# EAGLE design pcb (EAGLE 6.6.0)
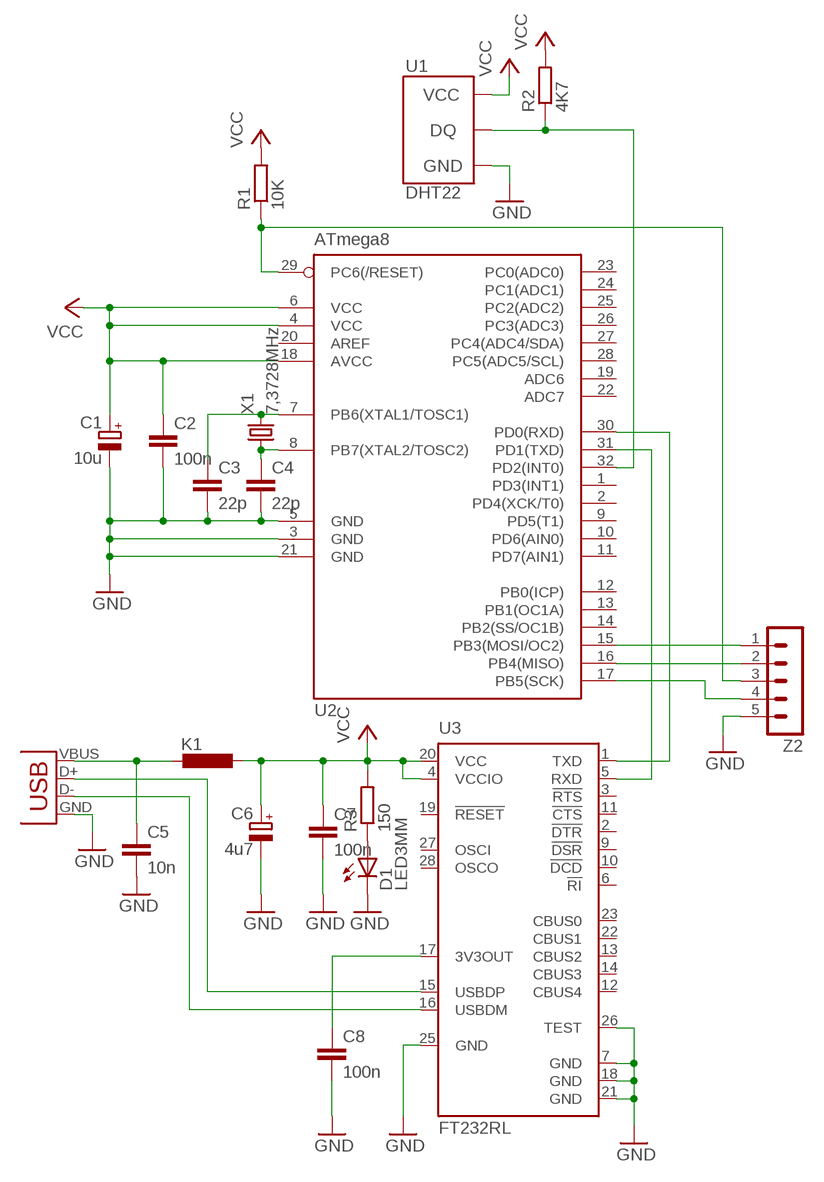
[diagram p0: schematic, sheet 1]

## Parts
C1  10u  CPOL-EUSMCA  [SMC_A]
C2  100n  C-EUC1206  [C1206]
C3  22p  C-EUC1206  [C1206]
C4  22p  C-EUC1206  [C1206]
C5  10n  C-EUC1206  [C1206]
C6  4u7  CPOL-EUSMCA  [SMC_A]
C7  100n  C-EUC1206  [C1206]
C8  100n  C-EUC1206  [C1206]
D1  LED3MM  [LED3MM]
K1  L-EU0805  [R0805]
R1  10K  R-EU_R1206  [R1206]
R2  4K7  R-EU_R1206  [R1206]
R3  150  R-EU_R1206  [R1206]
U1  DHT22  [DHT22]
U2  ATmega8  MEGA8-AI  [TQFP32-08]
U3  FT232RL  [SSOP28]
X1  7,3728MHz  CRYSTALHC49S  [HC49/S]
Z1  USB-A-H  [USB-A-H]
Z2  MA05-1  [MA05-1]

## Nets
CZ: R2.1 U1.2(DQ) U2.32(PD2(INT0))
GND: C1.- C2.2 C3.2 C4.2 C5.2 C6.- C7.2 C8.2 D1.K(C) U1.4(GND) U2.3(GND) U2.5(GND) U2.21(GND) U3.7(GND) U3.18(GND) U3.21(GND) U3.25(GND) U3.26(TEST) Z1.GND Z2.5
N$1: D1.A R3.1
N$2: C5.1 K1.2 Z1.VBUS
N$3: U3.15(USBDP) Z1.D+
N$4: U3.16(USBDM) Z1.D-
N$5: U2.17(PB5(SCK)) Z2.4
N$6: C8.1 U3.17(3V3OUT)
N$7: U2.30(PD0(RXD)) U3.1(TXD)
N$8: U2.31(PD1(TXD)) U3.5(RXD)
N$9: R1.1 U2.29(PC6(/RESET)) Z2.3
N$10: U2.16(PB4(MISO)) Z2.2
N$11: U2.15(PB3(MOSI/OC2)) Z2.1
N$33: C3.1 U2.7(PB6(XTAL1/TOSC1)) X1.2
N$34: C4.1 U2.8(PB7(XTAL2/TOSC2)) X1.1
VCC: C1.+ C2.1 C6.+ C7.1 K1.1 R1.2 R2.2 R3.2 U1.1(VCC) U2.4(VCC) U2.6(VCC) U2.18(AVCC) U3.4(VCCIO) U3.20(VCC)
Unconnected: U2.1(PD3(INT1)) U2.2(PD4(XCK/T0)) U2.9(PD5(T1)) U2.10(PD6(AIN0)) U2.11(PD7(AIN1)) U2.12(PB0(ICP)) U2.13(PB1(OC1A)) U2.14(PB2(SS/OC1B)) U2.19(ADC6) U2.20(AREF) U2.22(ADC7) U2.23(PC0(ADC0)) U2.24(PC1(ADC1)) U2.25(PC2(ADC2)) U2.26(PC3(ADC3)) U2.27(PC4(ADC4/SDA)) U2.28(PC5(ADC5/SCL)) U3.2(!DTR) U3.3(!RTS) U3.6(!RI) U3.9(!DSR) U3.10(!DCD) U3.11(!CTS) U3.12(CBUS4) U3.13(CBUS2) U3.14(CBUS3) U3.19(!RESET) U3.22(CBUS1) U3.23(CBUS0) U3.27(OSCI) U3.28(OSCO)

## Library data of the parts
C1 C6 = rcl:CPOL-EU: POLARIZED CAPACITOR, European symbol
C2-C5 C7 C8 = rcl:C-EU: CAPACITOR, European symbol
D1 = led:LED: LED
K1 = rcl:L-EU: INDUCTOR, European symbol
R1-R3 = rcl:R-EU_: RESISTOR, European symbol
U1 = sensors:DHT22
U2 = atmel:MEGA8: MICROCONTROLLER 8 Kbytes FLASH, 1 kbytes SRAM, 512 bytes EEPROM, USART, 6-channel 10 bit ADC, 2-channel 8 bit ADC Pin compatible with Atmega48, ATMega88, ATMega168 Source: avr.lbr
U3 = ftdichip:FT232R: Source: http://www.ftdichip.com/Documents/DataSheets/DS_FT232R_v104.pdf
X1 = crystal:CRYSTAL: CRYSTAL
Z1 = con-usb:USB: USB Connectors
Z2 = con-lstb:MA05-1: PIN HEADER

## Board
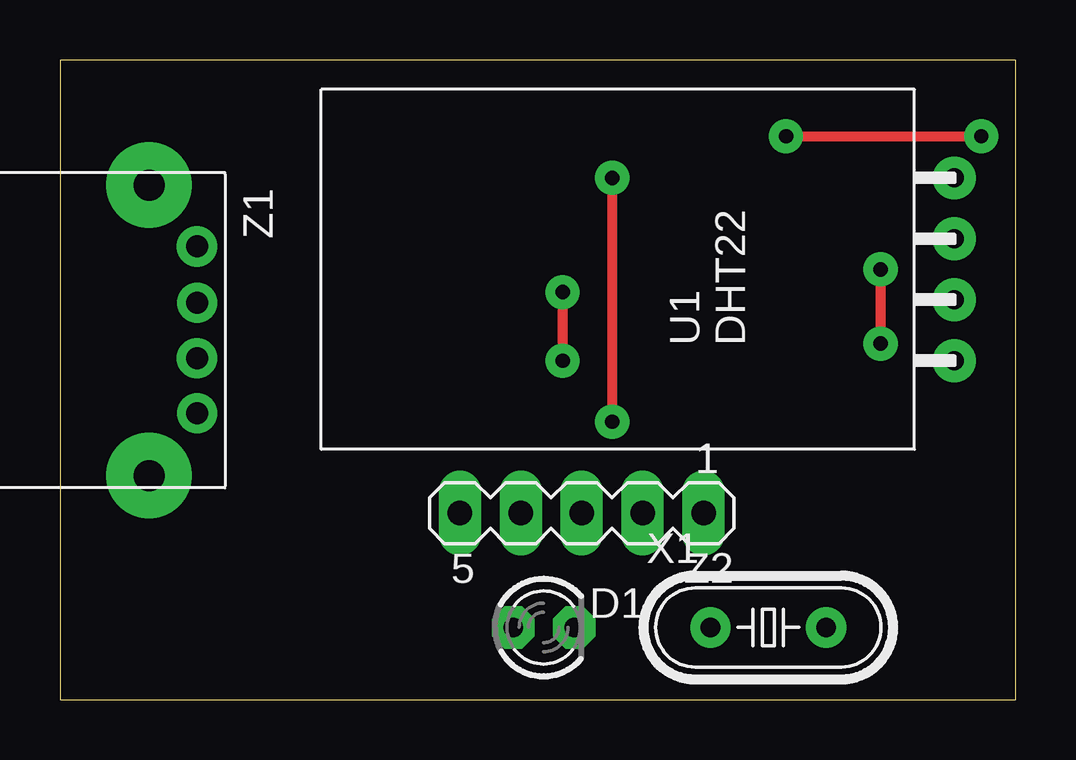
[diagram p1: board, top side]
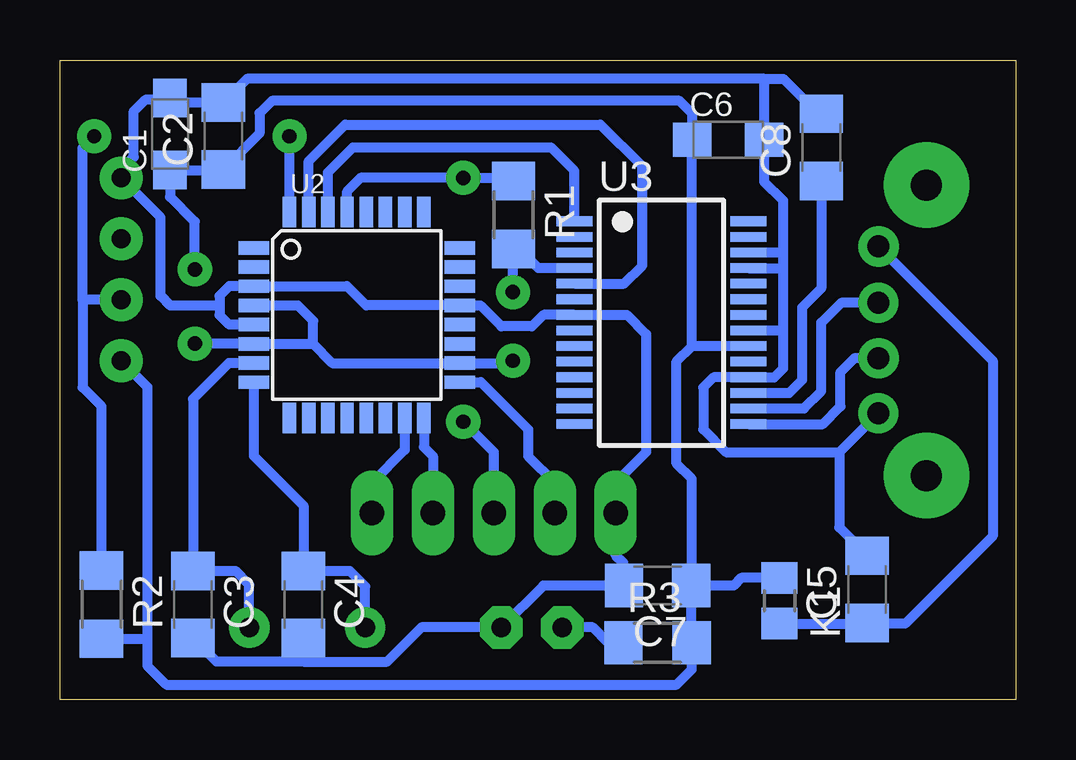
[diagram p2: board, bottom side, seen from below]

Size 39.83 x 26.66 mm. Coordinates in mm from the lower left corner, seen from the top.
Outline: 0,0 39.83,0 39.83,26.66 0,26.66 0,0
Copper layers (1*16): Top 0.035mm / dielectric 1.5mm / Bottom 0.035mm
Design rules "default": minimum track width 10mil, minimum drill 24mil, track to track 8mil, track to pad 8mil, pad to pad 8mil, via to via 8mil, smd to smd 8mil, copper to edge 40mil, drill to drill 8mil, minimum pad ring 10mil, minimum via ring 8mil, stop-mask expansion 4mil, vias tented up to drill 0mil, thermal gap 10mil

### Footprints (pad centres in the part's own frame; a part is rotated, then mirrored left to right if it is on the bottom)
SMC_A = smd 1.6 x 1.4: + -1.5,0; - 1.5,0
C1206 = smd 1.6 x 1.8: 1 -1.4,0; 2 1.4,0
LED3MM = drill 0.813 pad 1.778 octagon: A -1.27,0; K 1.27,0
R0805 = smd 1.3 x 1.5: 1 -0.95,0; 2 0.95,0
R1206 = smd 1.6 x 1.803: 1 -1.422,0; 2 1.422,0
DHT22 = drill 0.8 pad 1.778: 1 -3.81,-2.04; 2 -1.27,-2.04; 3 1.27,-2.04; 4 3.81,-2.04
TQFP32-08 = smd 1.27 x 0.559: 1 -4.293,2.8; 2 -4.293,2; 3 -4.293,1.2; 4 -4.293,0.4; 5 -4.293,-0.4; 6 -4.293,-1.2; 7 -4.293,-2; 8 -4.293,-2.8; 17 4.293,-2.8; 18 4.293,-2; 19 4.293,-1.2; 20 4.293,-0.4; 21 4.293,0.4; 22 4.293,1.2; 23 4.293,2; 24 4.293,2.8 | smd 0.559 x 1.27: 9 -2.8,-4.293; 10 -2,-4.293; 11 -1.2,-4.293; 12 -0.4,-4.293; 13 0.4,-4.293; 14 1.2,-4.293; 15 2,-4.293; 16 2.8,-4.293; 25 2.8,4.293; 26 2,4.293; 27 1.2,4.293; 28 0.4,4.293; 29 -0.4,4.293; 30 -1.2,4.293; 31 -2,4.293; 32 -2.8,4.293
SSOP28 = smd 0.4 x 1.5: 1 -4.225,-3.625; 2 -3.575,-3.625; 3 -2.925,-3.625; 4 -2.275,-3.625; 5 -1.625,-3.625; 6 -0.975,-3.625; 7 -0.325,-3.625; 8 0.325,-3.625; 9 0.975,-3.625; 10 1.625,-3.625; 11 2.275,-3.625; 12 2.925,-3.625; 13 3.575,-3.625; 14 4.225,-3.625; 15 4.225,3.625; 16 3.575,3.625; 17 2.925,3.625; 18 2.275,3.625; 19 1.625,3.625; 20 0.975,3.625; 21 0.325,3.625; 22 -0.325,3.625; 23 -0.975,3.625; 24 -1.625,3.625; 25 -2.275,3.625; 26 -2.925,3.625; 27 -3.575,3.625; 28 -4.225,3.625
HC49/S = drill 0.813 pad 1.676: 1 -2.413,0; 2 2.413,0
USB-A-H = drill 0.914 pad 1.676: D+ -0.002,-1.168; D- 0.008,1.143; GND 0.008,-3.458; VBUS -0.002,3.493 | drill 1.3 pad 3.556: P$5 -2,-6.056; P$6 -2,6.046
MA05-1 = drill 1.016 pad 1.778 long: 1 -5.08,0; 2 -2.54,0; 3 0,0; 4 2.54,0; 5 5.08,0

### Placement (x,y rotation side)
C1  35.24,23.57 90 bottom
C2  33.02,23.5 90 bottom
C3  34.29,3.97 270 bottom
C4  29.69,3.97 270 bottom
C5  6.19,4.6 90 bottom
C6  11.98,23.34 0 bottom
C7  14.92,4.76 180 bottom
C8  8.1,23.02 90 bottom
D1  20.16,3.02 0 top
K1  9.84,4.13 270 bottom
R1  20.93,20.2 270 bottom
R2  38.1,3.97 270 bottom
R3  14.92,2.38 0 bottom
U1  35.24,17.94 90 top
U2  27.46,16.03 0 bottom
U3  14.76,15.72 270 bottom
X1  29.53,3.02 0 top
Z1  5.71,15.4 0 top
Z2  21.75,7.78 180 top

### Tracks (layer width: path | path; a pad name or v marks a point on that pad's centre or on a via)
CZ  (via drill 0.6 pad 1.42)
  Top 0.406: v30.26,23.48 v38.41,23.48
  Bottom 0.406: R2.1 38.1,12.22 38.89,13.02 38.89,16.67 | U1.2 38.89,16.67 | 38.89,16.67 38.89,22.99 v38.41,23.48 | U2.32 v30.26,23.48 | v30.26,23.48
GND
  Bottom 0.406: 9.68,15.4 9.68,13.81 10.05,13.44 U3.18 12.59,13.44 13.02,13.02 13.02,11.27 12.06,10.32 7.34,10.32 | U3.21 9.69,15.39 9.68,15.4 | 9.68,15.4 9.68,18.1 | U3.25 9.79,17.99 9.68,18.1 | 33.84,2.09 C3.2 33.31,1.59 29.69,1.59 | C4.2 29.69,1.59 | 9.68,18.1 9.68,18.57 | 9.68,18.57 9.68,20.8 10.48,21.59 C6.- 10.48,25.88 | U3.26 9.75,18.64 9.68,18.57 | 29.69,1.59 26.19,1.59 24.77,3.02 D1.K 19.68,4.76 C7.2 16.35,4.79 16.35,5.71 16.67,6.03 Z2.5 16.67,9.05 15.4,10.32 15.4,15.24 16.2,16.04 U3.7 19.68,16.04 20.16,15.56 21.43,15.56 22.31,16.43 U2.21 27.07,16.43 27.87,17.23 U2.3 32.77,17.23 33.18,16.83 33.18,16.51 | U2.5 32.78,15.63 33.18,16.03 33.18,16.51 | 33.18,16.51 33.26,16.43 35.24,16.43 35.64,16.83 35.64,20.11 U1.4 37.28,22.09 36.75,22.62 36.75,24.53 36.27,25 35.25,25 C1.- | 10.48,25.88 32.04,25.88 C2.2 35.14,24.89 C1.- | 35.14,25.37 C1.- | C8.2 8.23,24.42 9.68,25.88 10.48,25.88 | 7.34,10.32 Z1.GND | 7.34,10.32 7.34,7.19 6.19,6.03 C5.2
N$1
  Bottom 0.406: R3.1 16.99,2.38 17.62,3.02 D1.A
N$2
  Bottom 0.406: Z1.VBUS 0.95,14.13 0.95,6.83 4.6,3.17 6.16,3.17 C5.1 6.22,3.18 K1.2
N$3
  Bottom 0.406: U3.15 8.04,11.49 7.3,12.22 7.3,13.65 6.72,14.23 Z1.D+
N$4
  Bottom 0.406: U3.16 8.81,12.14 8.1,12.86 8.1,15.72 7.27,16.54 Z1.D-
N$5
  Bottom 0.406: U2.17 22.28,13.23 20.32,11.27 20.32,10.16 19.21,9.05 Z2.4
N$6
  Bottom 0.406: U3.17 9.43,12.79 8.89,13.34 8.89,16.35 8.1,17.14 C8.1
N$7
  Bottom 0.406: U3.1 18.39,22.04 19.37,23.02 27.62,23.02 28.66,21.98 U2.30
N$8
  Bottom 0.406: U2.31 29.46,22.45 27.94,23.97 17.3,23.97 15.56,22.23 15.56,18.1 16.31,17.34 U3.5
N$9  (via drill 0.6 pad 1.42)
  Top 0.406: v23.02,21.75 v23.02,11.59
  Bottom 0.406: 20.64,21.91 20.56,21.99 R1.1 21.05,21.75 v23.02,21.75 27.3,21.75 27.86,21.19 U2.29 | Z2.3 21.75,10.32 v23.02,11.59
N$10
  Bottom 0.406: U2.16 24.66,10.54 24.29,10.16 Z2.2
N$11
  Bottom 0.406: U2.15 25.46,10.41 26.83,9.05 Z2.1
N$33
  Bottom 0.406: X1.2 31.94,4.79 32.52,5.37 C3.1 34.29,12.54 32.8,14.03 U2.7
N$34
  Bottom 0.406: X1.1 27.11,4.73 27.75,5.37 C4.1 29.69,8.1 31.76,10.17 U2.8
VCC  (via drill 0.6 pad 1.42)
  Top 0.406: v34.21,14.84 v34.21,17.94 | v20.95,16.99 v20.95,14.13
  Bottom 0.406: 13.81,2.53 R3.2 | 36.2,2.54 36.2,13.04 U1.1 | 36.2,2.54 36.2,1.43 35.4,0.64 14.13,0.64 13.49,1.27 R3.2 | R2.2 36.2,2.55 36.2,2.54 | U3.20 13.49,14.74 | 13.49,14.74 14.13,14.11 14.13,9.84 13.49,9.21 13.49,4.79 C7.1 | 13.49,14.74 13.49,23.32 C6.+ 13.49,23.35 13.49,24.45 14.01,24.96 31,24.96 31.51,24.45 31.51,23.6 C2.1 33.04,22.07 C1.+ 35.24,20.95 34.21,19.92 v34.21,17.94 | 29.28,14.83 28.48,14.03 U2.18 21.05,14.03 v20.95,14.13 | 29.28,14.83 U2.6 33.97,14.83 v34.21,14.84 | 29.28,14.83 29.28,15.79 29.93,16.43 U2.4 | C7.1 13.52,2.4 R3.2 | v20.95,16.99 20.95,18.75 R1.2 20.68,18.78 19.9,17.99 U3.4 | K1.1 11.43,5.08 11.75,4.76 C7.1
